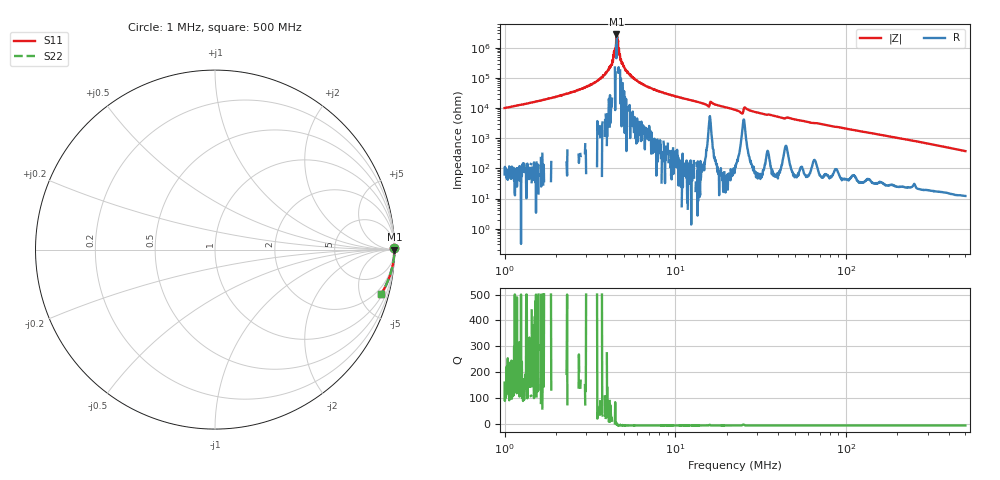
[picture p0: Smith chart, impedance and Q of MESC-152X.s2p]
!s-Parameter Generated by FASTRON Sdn. Bhd.
!FASTRON P/N : MESC-152X
!Keysight Technologies,E4991B,MY54100416,A.01.15
!Date: Fri Mar 27 13:11:57 2026
!Version  : Rev00 Fri Mar 27 13:11:57 2026
!Data & Calibration Information:
!PortZ  Port1:50+j0  Port2:50+j0
!When reading, reference impedance value at option line is always used.
! Remarks : This data is being provided solely for informational purposes.
!Freq	S11	S21	S12	S22
# Hz S dB R 50
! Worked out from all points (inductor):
!   1601 points, 1 MHz to 500 MHz, reference 50 ohm
!   read as one part in series: L = 1.52 mH near 1.032 MHz
!   highest |Z| = 2.77 Mohm at 4.513 MHz (marker M1)
!   self-resonance near 4.513 MHz
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1000000  -0.00 0.6  -40.06 -89.1  -40.06 -89.1  -0.00 0.6
1920401  0.00 0.3  -47.08 -90.0  -47.08 -90.0  0.00 0.3
2820919  0.00 0.1  -52.84 -90.3  -52.84 -90.3  0.00 0.1
3412295  0.00 0.1  -57.27 -90.1  -57.27 -90.1  0.00 0.1
3863901  -0.00 0.0  -62.16 -89.4  -62.16 -89.4  -0.00 0.0
4192277  -0.00 0.0  -68.58 -88.6  -68.58 -88.6  -0.00 0.0
4409396  0.00 0.0  -78.01 -96.9  -78.01 -96.9  0.00 0.0
4513363  -0.00 0.0  -88.86 -80.6  -88.86 -80.6  -0.00 0.0
4601872  0.00 -0.0  -82.86 122.9  -82.86 122.9  0.00 -0.0
4992965  -0.00 -0.0  -67.95 85.3  -67.95 85.3  -0.00 -0.0
5480788  -0.00 -0.0  -62.05 88.5  -62.05 88.5  -0.00 -0.0
6552974  -0.00 -0.1  -55.36 88.5  -55.36 88.5  -0.00 -0.1
7957584  -0.00 -0.2  -51.35 88.7  -51.35 88.7  -0.00 -0.2
1.534122e7  -0.00 -0.5  -41.91 87.2  -41.91 87.2  -0.00 -0.5
1.645218e7  -0.00 -0.4  -43.39 86.6  -43.39 86.6  -0.00 -0.4
2.236068e7  -0.00 -0.6  -38.92 88.8  -38.92 88.8  -0.00 -0.6
2.426102e7  -0.01 -0.8  -36.91 82.7  -36.91 82.7  -0.01 -0.8
2.601791e7  -0.01 -0.6  -39.71 84.4  -39.71 84.4  -0.01 -0.6
3.33604e7  -0.00 -0.9  -35.84 88.0  -35.84 88.0  -0.00 -0.9
6.307767e7  -0.01 -1.8  -30.18 86.3  -30.18 86.3  -0.01 -1.8
1.77937e8  -0.05 -4.9  -21.31 83.7  -21.31 83.7  -0.05 -4.9
5e8  -0.37 -14.9  -11.81 73.3  -11.81 73.3  -0.37 -14.9
